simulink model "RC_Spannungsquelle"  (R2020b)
settings: Solver=VariableStepAuto  StartTime=0.0  StopTime=10.0  RelTol=1e-3
model workspace (MAT data in the model file):
  C = 0.1
  R = 5
  Us = 12

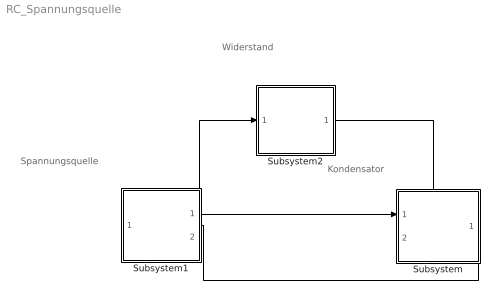
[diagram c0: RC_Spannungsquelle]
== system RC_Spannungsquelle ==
  note: Spannungsquelle
  note: Widerstand
  note: Kondensator
  Subsystem : Subsystem
  Subsystem1 : Subsystem
  Subsystem2 : Subsystem
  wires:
  Subsystem1/1(Us) -> Subsystem/1(Us)
  Subsystem/1(i_out) -> Subsystem1/1(i_in)
  Subsystem1/2(i_out) -> Subsystem2/1(i_in)
  Subsystem2/1(i_out) -> Subsystem/2(i_in)

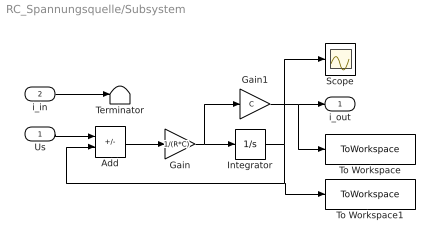
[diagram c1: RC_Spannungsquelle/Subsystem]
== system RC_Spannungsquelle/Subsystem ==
  Us : Inport
  i_in : Inport  Port=2
  Add : Sum  Inputs=+-
  Gain : Gain  Gain=1/(R*C)
  Gain1 : Gain  Gain=C
  Integrator : Integrator
  Scope : Scope
  Terminator : Terminator
  To Workspace : ToWorkspace  VariableName=i  SaveFormat=Timeseries  SampleTime=-1
  To Workspace1 : ToWorkspace  VariableName=Uc  SaveFormat=Timeseries  SampleTime=-1
  i_out : Outport
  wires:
  Gain/1 -> Gain1/1, Integrator/1
  Integrator/1 -> Scope/1, Add/2, To Workspace1/1
  Us/1 -> Add/1
  Add/1 -> Gain/1
  Gain1/1 -> To Workspace/1, i_out/1
  i_in/1 -> Terminator/1

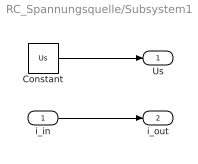
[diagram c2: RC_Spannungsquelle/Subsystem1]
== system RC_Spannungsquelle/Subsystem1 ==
  i_in : Inport
  Constant : Constant  Value=Us
  Us : Outport
  i_out : Outport  Port=2
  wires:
  Constant/1 -> Us/1
  i_in/1 -> i_out/1

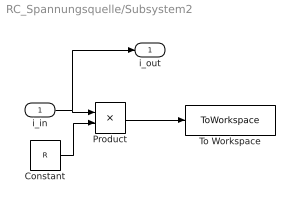
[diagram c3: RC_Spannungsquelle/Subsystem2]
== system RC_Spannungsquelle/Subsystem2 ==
  i_in : Inport
  Constant : Constant  Value=R
  Product : Product
  To Workspace : ToWorkspace  VariableName=Ur  SaveFormat=Timeseries  SampleTime=-1
  i_out : Outport
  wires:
  i_in/1 -> i_out/1, Product/1
  Constant/1 -> Product/2
  Product/1 -> To Workspace/1
